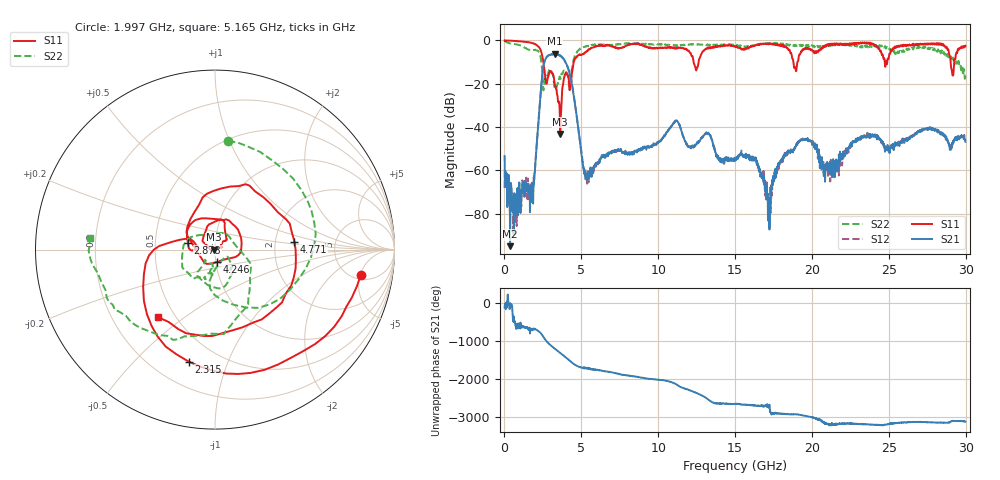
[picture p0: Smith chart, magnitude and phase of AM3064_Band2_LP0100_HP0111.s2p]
# Hz S DB R 50.0
!freq dBS11 angS11 dBS21 angS21 dBS12 angS12 dBS22 angS22
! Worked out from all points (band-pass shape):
!   1600 points, 10 MHz to 29.98 GHz, reference 50 ohm
!   highest |S21| = -6.14 dB at 3.271 GHz (marker M1); lowest = -94.9 dB at 366.1 MHz (marker M2)
!   |S21| within 3 dB of the highest: 2.636 GHz to 3.895 GHz (1.258 GHz wide, 38.5 % of centre)
!   lowest |S11| = -43.1 dB at 3.628 GHz (marker M3), VSWR 1.01, Z = 49.3 - j0.00473 ohm
!   |S11| at or under -10 dB: 2.537 GHz to 4.511 GHz (1.974 GHz wide, 56 % of centre); 12.31 GHz to 12.63 GHz (322 MHz wide, 2.58 % of centre); 18.8 GHz to 19.05 GHz (253.9 MHz wide, 1.34 % of centre)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
!   |S22| runs from -23.1 to -0.2 dB; largest |S21 - S12| = 0.016
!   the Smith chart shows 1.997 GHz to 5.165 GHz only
!   S11 on the Smith chart (normalised r, x): 1.997 GHz: 5.80, -5.11; 2.315 GHz: 0.35, -0.74; 2.878 GHz: 0.73, +0.06; 4.246 GHz: 1.01, -0.14; 4.771 GHz: 2.56, +0.29; 5.165 GHz: 0.40, -0.40
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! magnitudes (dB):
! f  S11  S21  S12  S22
! 10 MHz  0.0  -53.4  -68.0  -0.2
! 366.1 MHz  -0.1  -94.9  -75.8  -1.4
! 1.697 GHz  -1.0  -69.3  -73.0  -4.5
! 1.997 GHz  -1.7  -58.0  -57.7  -4.3
! 2.315 GHz  -3.9  -27.7  -27.6  -6.9
! 2.878 GHz  -16.1  -6.8  -6.8  -14.2
! 3.271 GHz  -19.7  -6.1  -6.2  -22.1
! 3.628 GHz  -43.1  -7.1  -7.0  -17.4
! 4.246 GHz  -22.9  -15.3  -15.4  -19.8
! 4.771 GHz  -7.0  -39.1  -38.6  -4.9
! 5.015 GHz  -6.7  -53.2  -52.1  -3.6
! 5.165 GHz  -6.2  -59.1  -60.1  -3.1
! 10 GHz  -3.5  -47.2  -47.2  -1.8
! 11.16 GHz  -3.5  -37.2  -36.9  -2.4
! 15 GHz  -2.7  -54.5  -54.0  -1.9
! 16.32 GHz  -2.2  -55.4  -54.8  -2.2
! 17.24 GHz  -1.5  -87.3  -74.8  -1.4
! 18.17 GHz  -2.4  -54.3  -53.3  -2.2
! 19.99 GHz  -4.4  -47.0  -46.8  -2.2
! 21.17 GHz  -1.7  -61.5  -58.0  -1.9
! 25 GHz  -8.1  -49.4  -51.3  -3.4
! 29.98 GHz  -2.4  -46.7  -45.9  -15.8
